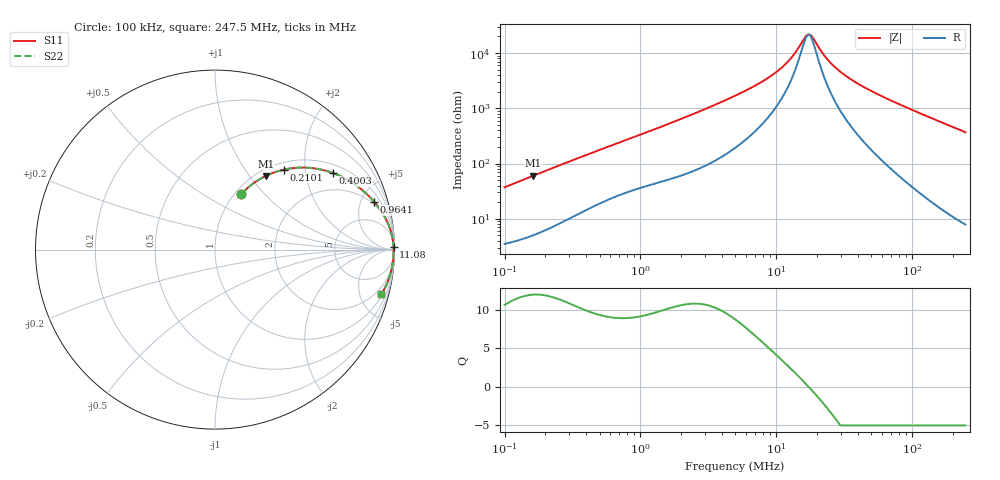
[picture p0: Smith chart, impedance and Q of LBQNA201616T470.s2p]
! LBQNA201616T470  S-PARAMETER MODEL  ( General Type )
! Model Generated by TAIYO YUDEN Corporation (http://www.ty-top.com)
! Version 1.0
! TAIYO YUDEN Control No. 191025NI43SB-FBB
! Copyright(c) 2019 TAIYO YUDEN CO.,LTD. All Rights Reserved.
! Product Description (link to TY-COMPAS)
! https://ds.yuden.co.jp/TYCOMPAS/or/detail?pn=LBQNA201616T470K&u=M
! Products Name : Inductors
! Characteristics :
!  Inductance : 47 uH , SRF(min) : 11 MHz , DC Resistance(max) : 3.12 Ohm
!  Rated Current : Saturation :110 mA , Temp Rise : 120 mA (20 degC)
!  Case Size : 2.0 x 1.6 / 0.079 x 0.063 [mm/inch] , Thickness : 1.6 / 0.063 [mm/inch]
!  (Conditions: Temperature = 25 degC , DC Bias Current/Voltage = 0A / 0V)
! External Node Assignments :
!  1  o---GGG---o  2
! GND o---------o GND
! Frequency Range : 0.1MHz  -  247.502633MHz  [ 402 STEP ]
# MHz S RI R 50
! Freq[MHz].  S11 Real  S11 Imag  S21 Real  S21 Imag  S12 Real  S12 Imag  S22 Real  S22 Imag
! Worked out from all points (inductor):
!   401 points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, 100 kHz to 247.5 MHz, reference 50 ohm
!   read as one part in series: L = 59 uH near 104 kHz
!   highest Q = 11.9 at 163 kHz (marker M1), where L = 58.8 uH
!   self-resonance near 17.03 MHz
!   S11 on the Smith chart (normalised r, x): 100 kHz: 1.07, +0.74; 210.1 kHz: 1.13, +1.54; 400.3 kHz: 1.29, +2.85; 964.1 kHz: 1.70, +6.38; 11.08 MHz: open; 247.5 MHz: 1.16, -7.38
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0.1  0.1442 0.3072  0.8558 -0.3072  0.8558 -0.3072  0.1442 0.3072
0.162967  0.2833 0.4106  0.7167 -0.4106  0.7167 -0.4106  0.2833 0.4106
0.210083  0.3841 0.4457  0.6159 -0.4457  0.6159 -0.4457  0.3841 0.4457
0.37019  0.6272 0.4366  0.3728 -0.4366  0.3728 -0.4366  0.6272 0.4366
0.400277  0.6574 0.4266  0.3426 -0.4266  0.3426 -0.4266  0.6574 0.4266
0.615187  0.7942 0.3524  0.2058 -0.3524  0.2058 -0.3524  0.7942 0.3524
0.964136  0.8875 0.2656  0.1125 -0.2656  0.1125 -0.2656  0.8875 0.2656
1.370406  0.9333 0.2034  0.0667 -0.2034  0.0667 -0.2034  0.9333 0.2034
2.71511  0.9771 0.11  0.0229 -0.11  0.0229 -0.11  0.9771 0.11
4.974964  0.9899 0.0581  0.0101 -0.0581  0.0101 -0.0581  0.9899 0.0581
7.950688  0.9935 0.0316  0.00655 -0.0316  0.00655 -0.0316  0.9935 0.0316
11.08235  0.9947 0.0171  0.00535 -0.0171  0.00535 -0.0171  0.9947 0.0171
13.21257  0.995 0.0102  0.00495 -0.0102  0.00495 -0.0102  0.995 0.0102
16.70301  0.9954 0.00139  0.00463 -0.00139  0.00463 -0.00139  0.9954 0.00139
17.36851  0.9954 -6.6e-05  0.00459 6.6e-05  0.00459 6.6e-05  0.9954 -6.6e-05
18.41681  0.9955 -0.00226  0.00455 0.00226  0.00455 0.00226  0.9955 -0.00226
23.28209  0.9955 -0.0112  0.00451 0.0112  0.00451 0.0112  0.9955 -0.0112
29.43265  0.9953 -0.0208  0.0047 0.0208  0.0047 0.0208  0.9953 -0.0208
41.83506  0.9944 -0.0376  0.00559 0.0376  0.00559 0.0376  0.9944 -0.0376
68.1772  0.991 -0.0691  0.00898 0.0691  0.00898 0.0691  0.991 -0.0691
132.4626  0.9757 -0.139  0.0243 0.139  0.0243 0.139  0.9757 -0.139
247.5026  0.9271 -0.2495  0.0729 0.2495  0.0729 0.2495  0.9271 -0.2495
